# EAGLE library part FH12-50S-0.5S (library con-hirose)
0.5mm Pitch Connectors For FPC/FFC Source: Data sheet
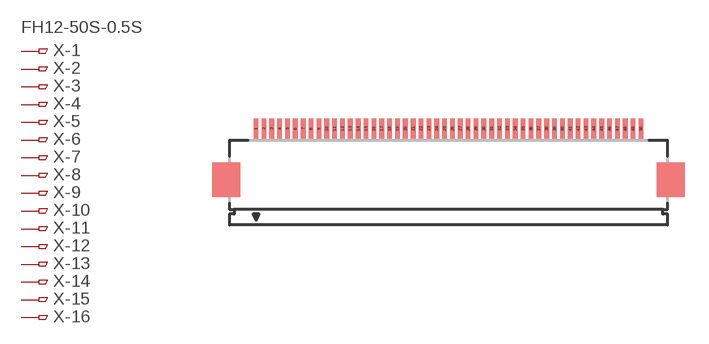
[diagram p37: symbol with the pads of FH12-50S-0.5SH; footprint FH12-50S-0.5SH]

Designator prefix X; gates -1=PINV -2=PIN -3=PIN -4=PIN -5=PIN -6=PIN -7=PIN -8=PIN -9=PIN -10=PIN -11=PIN -12=PIN -13=PIN -14=PIN -15=PIN -16=PIN -17=PIN -18=PIN -19=PIN -20=PIN -21=PIN -22=PIN -23=PIN -24=PIN -25=PIN -26=PIN -27=PIN -28=PIN -29=PIN -30=PIN -31=PIN -32=PIN -33=PIN -34=PIN -35=PIN -36=PIN -37=PIN -38=PIN -39=PIN -40=PIN -41=PIN -42=PIN -43=PIN -44=PIN -45=PIN -46=PIN -47=PIN -48=PIN -49=PIN -50=PIN

## FH12-50S-0.5SH (MPN: FH12-50S-0.5SH(55); OC_FARNELL: 1324557; OC_NEWARK: 34M6181)  [FH12-50S-0.5SH]
1  -1:1  pas
2  -2:1  pas
3  -3:1  pas
4  -4:1  pas
5  -5:1  pas
6  -6:1  pas
7  -7:1  pas
8  -8:1  pas
9  -9:1  pas
10  -10:1  pas
11  -11:1  pas
12  -12:1  pas
13  -13:1  pas
14  -14:1  pas
15  -15:1  pas
16  -16:1  pas
17  -17:1  pas
18  -18:1  pas
19  -19:1  pas
20  -20:1  pas
21  -21:1  pas
22  -22:1  pas
23  -23:1  pas
24  -24:1  pas
25  -25:1  pas
26  -26:1  pas
27  -27:1  pas
28  -28:1  pas
29  -29:1  pas
30  -30:1  pas
31  -31:1  pas
32  -32:1  pas
33  -33:1  pas
34  -34:1  pas
35  -35:1  pas
36  -36:1  pas
37  -37:1  pas
38  -38:1  pas
39  -39:1  pas
40  -40:1  pas
41  -41:1  pas
42  -42:1  pas
43  -43:1  pas
44  -44:1  pas
45  -45:1  pas
46  -46:1  pas
47  -47:1  pas
48  -48:1  pas
49  -49:1  pas
50  -50:1  pas

## Footprint FH12-50S-0.5SH (pad centres in mm)
0.5mm Pitch Connectors For FPC/FFC Source: Data sheet
smd 0.3 x 1.3: 1 -12.25,3.25; 2 -11.75,3.25; 3 -11.25,3.25; 4 -10.75,3.25; 5 -10.25,3.25; 6 -9.75,3.25; 7 -9.25,3.25; 8 -8.75,3.25; 9 -8.25,3.25; 10 -7.75,3.25; 11 -7.25,3.25; 12 -6.75,3.25; 13 -6.25,3.25; 14 -5.75,3.25; 15 -5.25,3.25; 16 -4.75,3.25; 17 -4.25,3.25; 18 -3.75,3.25; 19 -3.25,3.25; 20 -2.75,3.25; 21 -2.25,3.25; 22 -1.75,3.25; 23 -1.25,3.25; 24 -0.75,3.25; 25 -0.25,3.25; 26 0.25,3.25; 27 0.75,3.25; 28 1.25,3.25; 29 1.75,3.25; 30 2.25,3.25; 31 2.75,3.25; 32 3.25,3.25; 33 3.75,3.25; 34 4.25,3.25; 35 4.75,3.25; 36 5.25,3.25; 37 5.75,3.25; 38 6.25,3.25; 39 6.75,3.25; 40 7.25,3.25; 41 7.75,3.25; 42 8.25,3.25; 43 8.75,3.25; 44 9.25,3.25; 45 9.75,3.25; 46 10.25,3.25; 47 10.75,3.25; 48 11.25,3.25; 49 11.75,3.25; 50 12.25,3.25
